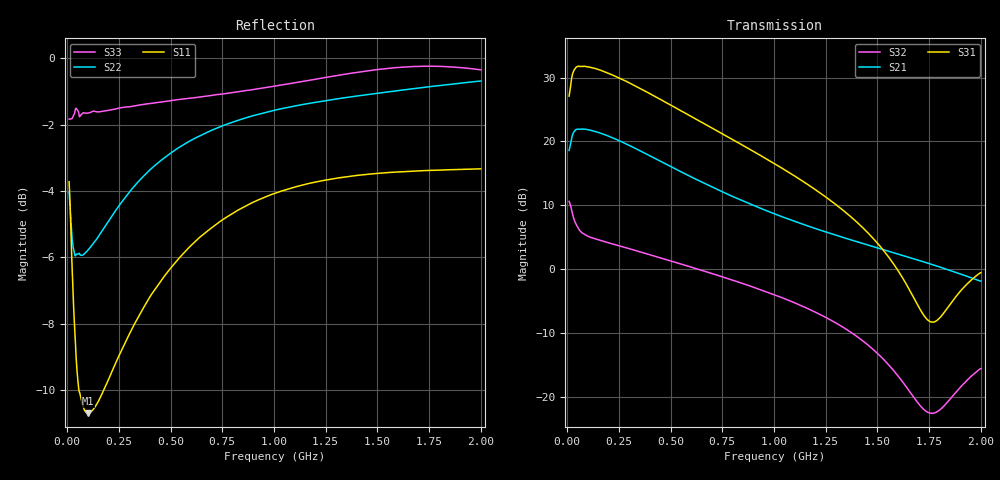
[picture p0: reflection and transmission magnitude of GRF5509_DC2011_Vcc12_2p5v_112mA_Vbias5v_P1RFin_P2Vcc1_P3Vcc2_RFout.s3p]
!Keysight Technologies,N5244B,MY57181157,A.18.40.03
!Date: Wednesday, April 29, 2026 14:33:57
!Correction: S11(C  3-Port  )
!S12(C  3-Port  )
!S13(C  3-Port  )
!S21(C  3-Port  )
!S22(C  3-Port  )
!S23(C  3-Port  )
!S31(C  3-Port  )
!S32(C  3-Port  )
!S33(C  3-Port  )
!S3P File: Measurements: <S11,S12,S13>,
!<S21,S22,S23>,
!<S31,S32,S33>:
# Hz S  dB  R 50
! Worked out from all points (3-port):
!   1991 points, 10 MHz to 2 GHz, reference 50 ohm
!   strongest paths, dB at 10 MHz, 507 MHz, 1.005 GHz, 1.503 GHz, 2 GHz:
!     S31: 27.1, 25.6, 16.5, 3.9, -0.6
!     S21: 18.6, 16.0, 8.6, 3.3, -1.9
!     S32: 10.6, 1.2, -4.1, -13.3, -15.6
!   lowest |S11| = -10.7 dB at 102 MHz (marker M1), VSWR 1.82, Z = 31.7 - j15.9 ohm
!   |S11| at or under -10 dB: 57.21 MHz to 177.1 MHz (119.9 MHz wide, 102 % of centre)
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1e7  -3.72 -52.1  -22.16 -33.9  -58.12 -142.4
     18.58 -136.3  -4.03 -77.2  -32.72 -85.8
     27.09 76.4  10.59 -175.6  -1.83 -118.6
3e7  -7.22 -88.0  -26.55 -42.5  -64.42 110.1
     21.30 -161.6  -5.71 -121.2  -43.46 146.0
     30.88 31.4  8.18 160.8  -1.74 -151.1
4.3e7  -8.91 -103.8  -28.50 -42.3  -65.11 -56.1
       21.85 -172.1  -5.92 -134.8  -43.11 -26.5
       31.59 16.4  7.08 157.5  -1.51 -160.0
1.02e8  -10.70 -127.9  -32.19 -30.3  -71.80 -57.8
        21.82 163.7  -5.77 -155.0  -50.85 33.8
        31.67 -16.2  5.12 153.2  -1.65 -170.5
1.68e8  -10.12 -134.5  -33.19 -24.0  -70.26 73.2
        21.22 146.5  -5.21 -159.8  -45.48 46.2
        31.07 -37.9  4.41 146.5  -1.60 -173.0
2.46e8  -9.03 -137.6  -33.61 -21.4  -66.68 87.6
        20.19 130.0  -4.49 -162.7  -42.63 44.3
        30.02 -58.4  3.69 137.7  -1.50 -173.8
4.72e8  -6.55 -144.5  -34.45 -23.2  -60.55 83.6
        16.54 95.8  -2.99 -170.4  -39.81 33.9
        26.21 -103.6  1.54 113.8  -1.30 -173.9
6.73e8  -5.23 -150.3  -35.29 -25.6  -58.01 83.8
        13.28 76.1  -2.24 -176.1  -39.18 29.7
        22.59 -133.5  -0.43 95.5  -1.14 -173.6
1.005e9  -4.07 -159.0  -36.47 -27.6  -54.55 84.8
         8.61 55.2  -1.56 177.2  -39.55 30.5
         16.46 -172.7  -4.07 68.6  -0.83 -173.8
2e9  -3.33 -177.6  -39.28 -44.4  -48.18 93.4
     -1.90 11.3  -0.68 156.3  -34.82 70.6
     -0.58 -126.5  -15.60 121.6  -0.34 172.3
